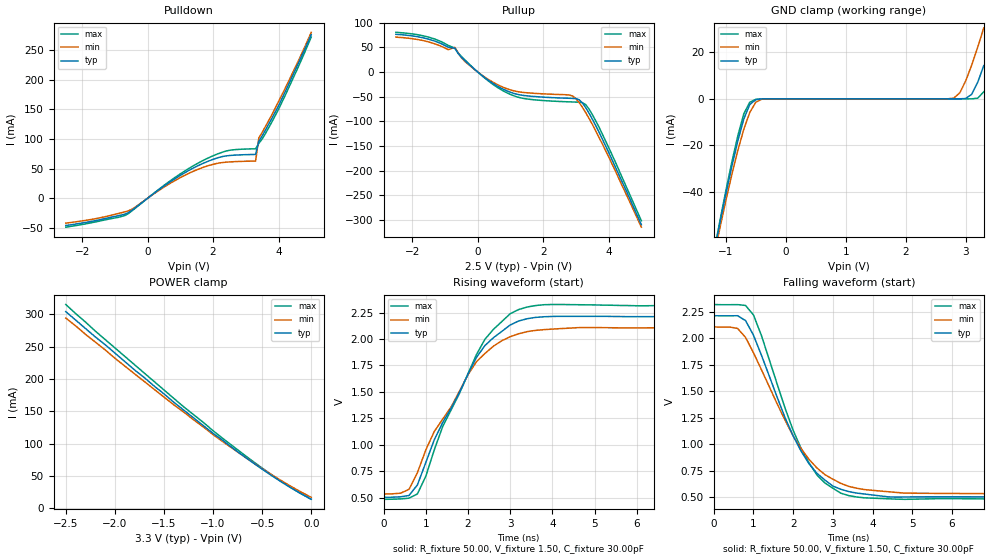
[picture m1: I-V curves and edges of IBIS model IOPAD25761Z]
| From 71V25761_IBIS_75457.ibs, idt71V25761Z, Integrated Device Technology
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|IOIN   NC   NC   NC   NC
|OC   NC   NC   NC   NC
|IN   NC   NC   NC   NC
|CLK   NC   NC   NC   NC
|   Model IOPAD25761Z
[Model]   IOPAD25761Z
Model_type   I/O
Polarity   Non-Inverting
Enable   Active-High
Vinl =  0.700V
Vinh =  1.700V
Vmeas =  1.250V
Vref = 1.50   | AC Test Load
Rref = 50.00   |  as shown in
Cref = 0.00pF   |  the datasheet
C_comp   1.56pF   1.56pF   1.56pF
[Temperature Range]   25.00   70.00   0.000
[Pullup Reference]   2.50V   2.37V   2.62V
[Pulldown Reference]   0.000V   0.000V   0.000V
[POWER Clamp Reference]   3.30V   3.13V   3.46V
[GND Clamp Reference]   0.000V   0.000V   0.000V
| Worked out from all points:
|   slope of the pulldown table from 0 to 0.375 V, typ, clamps not added: 24.1 ohm
|   slope of the pullup table from 0 to 0.375 V, typ, clamps not added: 19.7 ohm
|   GND clamp passes 1 mA (typ) near -0.53 V on its own axis
|   rising waveform, R_fixture 50.00, V_fixture 1.50, C_fixture 30.00pF: 20-80 % time 1.27ns typ, 1.32ns min, 1.22ns max; typ from 0.502 V to 2.21 V
|   falling waveform, R_fixture 50.00, V_fixture 1.50, C_fixture 30.00pF: 20-80 % time 1.19ns typ, 1.33ns min, 1.1ns max; typ from 2.21 V to 0.501 V
[Pulldown]
| voltage   I(typ)   I(min)   I(max)
-2.5V     -46mA      -42mA      -48.8mA
-700mV    -26.97mA   -23.12mA   -29.28mA
-400mV    -17.03mA   -15.7mA    -17.88mA
800mV     31.66mA    28.72mA    33.64mA
1.7V      58.99mA    52.1mA     63.84mA
2.4V      71.42mA    60.84mA    79.71mA
3.3V      73.93mA    62.76mA    83.46mA
3.4V      96.36mA    102mA      92.66mA
3.6V      115mA      121mA      109mA
4V        156mA      163mA      150mA
4.6V      227mA      231mA      221mA
5V        276mA      280mA      272mA
[Pullup]
| voltage   I(typ)   I(min)   I(max)
-2.5V     76.6mA     70.8mA     80.6mA
-1.5V     66.65mA    61.1mA     70.82mA
-900mV    50.26mA    45.38mA    53.97mA
-700mV    48.54mA    50.16mA    48.58mA
-400mV    23.69mA    21.99mA    25.15mA
100mV     -5.468mA   -4.964mA   -5.877mA
1.1V      -43.33mA   -38.13mA   -48.19mA
2.9V      -53.55mA   -48.79mA   -60.79mA
3.2V      -62.75mA   -71.73mA   -62.34mA
3.5V      -95.5mA    -106mA     -86.2mA
4V        -163mA     -172mA     -153mA
5V        -310mA     -315mA     -302mA
[GND_clamp]
| voltage   I(typ)   I(min)   I(max)
-2.5V     -254mA     -248mA     -257mA
-1.2V     -66.68mA   -68.09mA   -66.18mA
-1.1V     -53.57mA   -55.7mA    -52.65mA
-900mV    -29.07mA   -32.6mA    -27.25mA
-700mV    -8.681mA   -13.05mA   -6.453mA
-600mV    -2.453mA   -5.846mA   -1.446mA
-500mV    -350uA     -1.468mA   -224uA
-300mV    -1.604uA   -8.507uA   -592nA
2.8V      711nA      298uA      31.43nA
2.9V      9.085uA    2.585mA    92.87nA
3.1V      1.972mA    14.54mA    15.51uA
3.3V      14.24mA    30.45mA    3.029mA
[POWER_clamp]
| voltage   I(typ)   I(min)   I(max)
-2.5V     304mA      294mA      315mA
-2.2V     265mA      257mA      274mA
-1.8V     214mA      208mA      222mA
-1.3V     152mA      149mA      157mA
-1V       116mA      114mA      120mA
-700mV    82.05mA    81.89mA    84.75mA
-400mV    50.33mA    51.76mA    51.65mA
-200mV    31.13mA    33.47mA    31.6mA
0V        14.24mA    17.13mA    14.01mA
[Ramp]
| variable   typ   min   max
dV/dt_r   1.04/0.90n   0.95/0.97n   1.12/0.81n
dV/dt_f   0.99/0.56n   0.91/0.67n   1.07/0.51n
R_load = 50.00
[Rising Waveform]
R_fixture = 50.00
V_fixture = 1.50
C_fixture = 30.00pF
R_dut = 0.75
L_dut = 0.10nH
C_dut = 0.53pF
| time   V(typ)   V(min)   V(max)
0s        502mV      533mV      483mV
600ps     519mV      577mV      494mV
800ps     619mV      735mV      534mV
1.2ns     1.047V     1.125V     951mV
1.4ns     1.21V      1.242V     1.172V
2ns       1.668V     1.663V     1.672V
2.4ns     1.938V     1.863V     1.997V
3ns       2.133V     2.022V     2.24V
3.4ns     2.192V     2.07V      2.303V
19.8ns    2.215V     2.109V     2.32V
[Falling Waveform]
R_fixture = 50.00
V_fixture = 1.50
C_fixture = 30.00pF
R_dut = 0.75
L_dut = 0.10nH
C_dut = 0.53pF
| time   V(typ)   V(min)   V(max)
0s        2.215V     2.109V     2.321V
600ps     2.215V     2.095V     2.32V
800ps     2.169V     2.01V      2.312V
1ns       2.031V     1.865V     2.222V
1.8ns     1.247V     1.225V     1.337V
2.2ns     935mV      959mV      961mV
2.8ns     662mV      713mV      634mV
3.4ns     553mV      602mV      515mV
5.2ns     503mV      537mV      483mV
19.8ns    501mV      533mV      483mV
